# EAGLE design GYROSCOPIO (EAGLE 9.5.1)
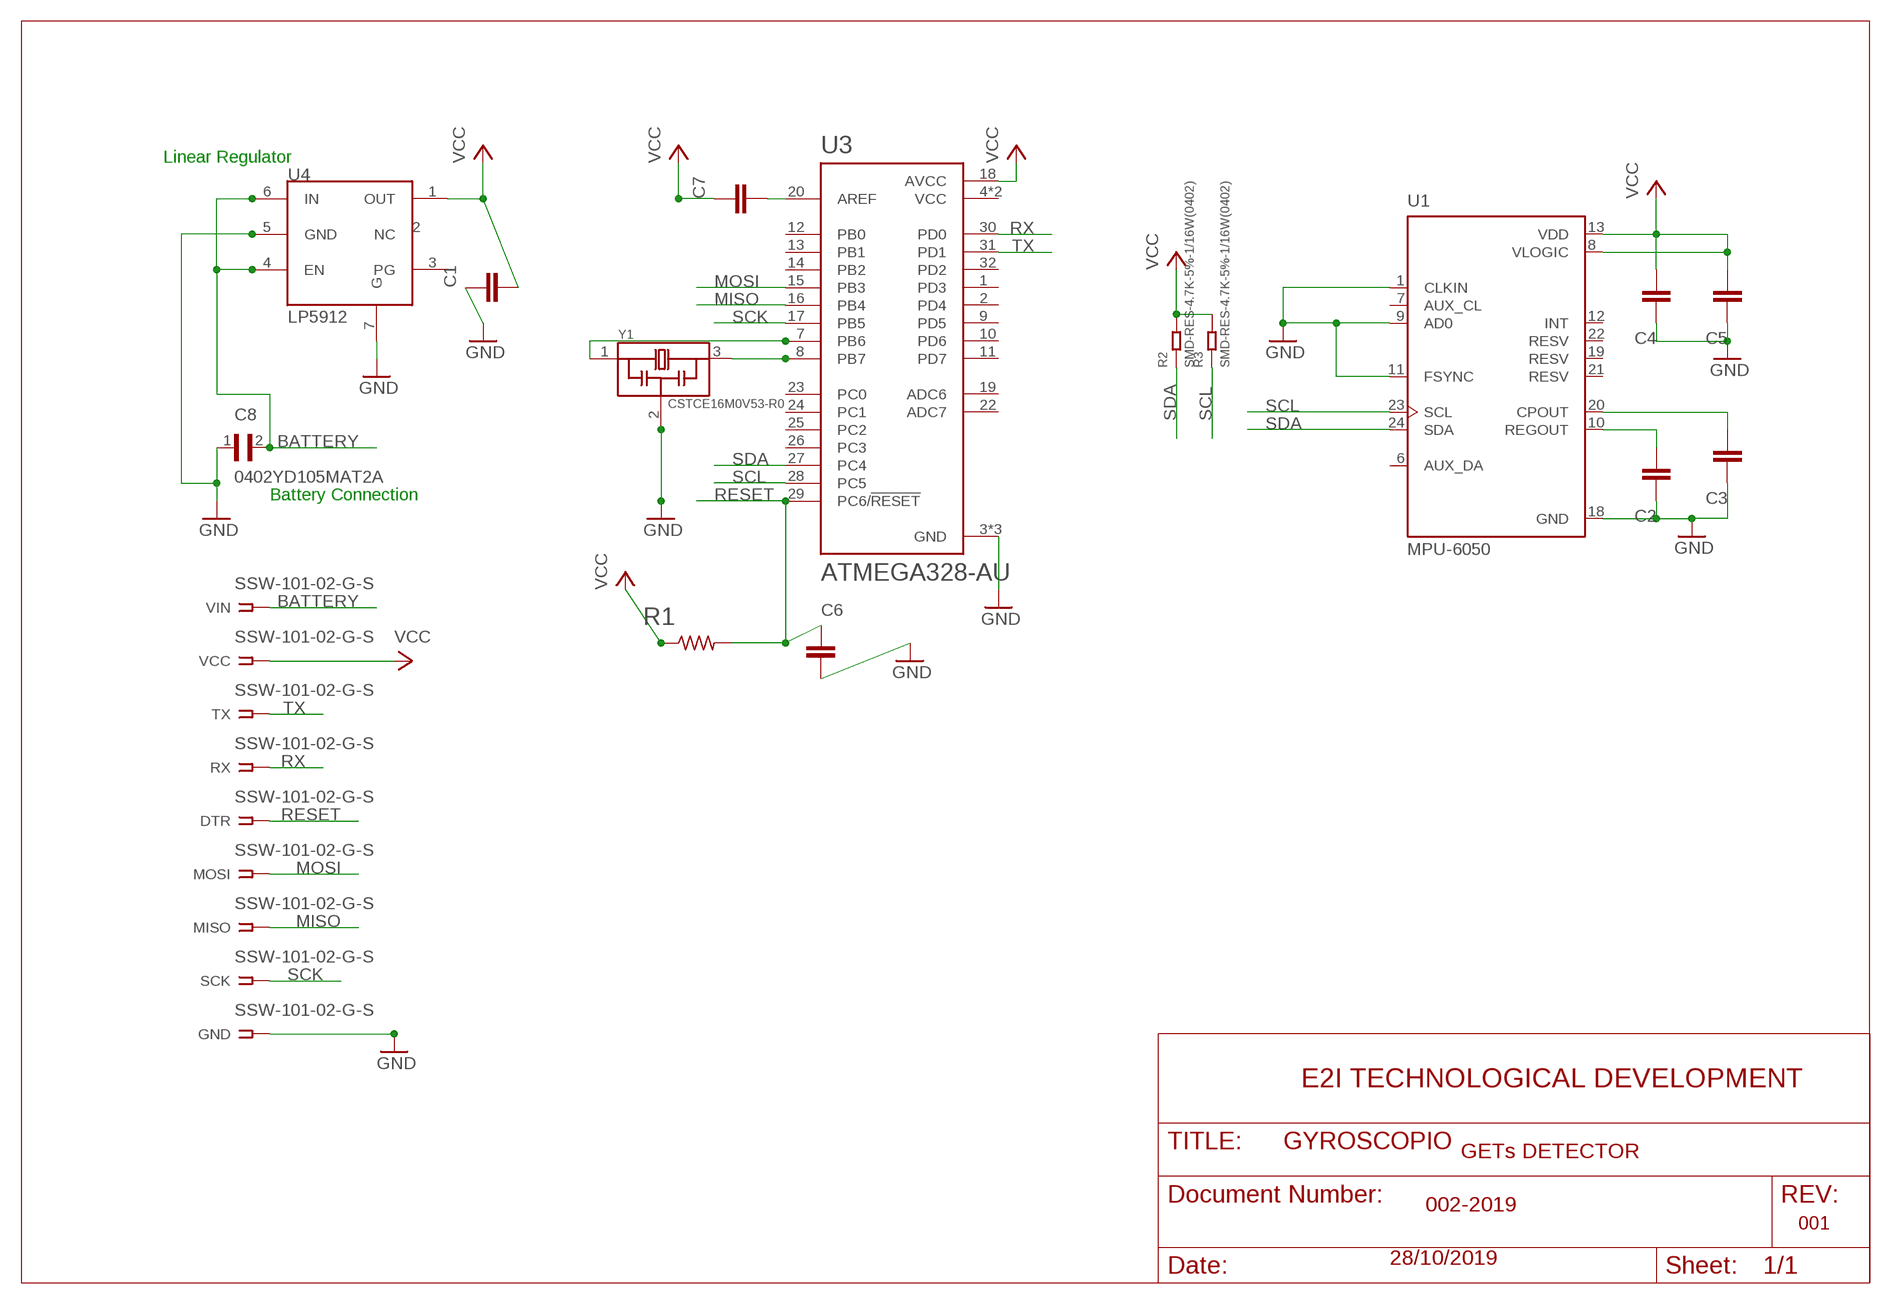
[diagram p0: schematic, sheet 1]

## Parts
C1  C-EUC0603  [C0603]
C2  C-EUC0603  [C0603]
C3  C-EUC0603  [C0603]
C4  C-EUC0603  [C0603]
C5  C-EUC0603  [C0603]
C6  C-EUC0603  [C0603]
C7  C-EUC0603  [C0603]
C8  0402YD105MAT2A  [CAPC1005X71N]
DTR  SSW-101-02-G-S  [SSW-101-02-G-S]
GND  SSW-101-02-G-S  [SSW-101-02-G-S]
MISO  SSW-101-02-G-S  [SSW-101-02-G-S]
MOSI  SSW-101-02-G-S  [SSW-101-02-G-S]
R1  R-US_R0603  [R0603]
R2  SMD-RES-4.7K-5%-1/16W(0402)  [R0402]
R3  SMD-RES-4.7K-5%-1/16W(0402)  [R0402]
RX  SSW-101-02-G-S  [SSW-101-02-G-S]
SCK  SSW-101-02-G-S  [SSW-101-02-G-S]
TX  SSW-101-02-G-S  [SSW-101-02-G-S]
U1  MPU-6050  [QFN50P400X400X95-24N]
U3  ATMEGA328-AU  [QFP80P900X900X120-32N]
U4  LP5912  [LP5912]
VCC  SSW-101-02-G-S  [SSW-101-02-G-S]
VIN  SSW-101-02-G-S  [SSW-101-02-G-S]
Y1  CSTCE16M0V53-R0  [OSC_CSTCE16M0V53-R0]

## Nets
BATTERY: C8.2 U4.4(EN) U4.6(IN) VIN.1
GND: C1.1 C2.1 C3.1 C4.1 C5.1 C6.2 C8.1 GND.1 U1.1(CLKIN) U1.9(AD0) U1.11(FSYNC) U1.18(GND) U3.3(GND) U3.5(GND) U3.21(GND) U4.5(GND) U4.7(G) Y1.2
MISO: MISO.1 U3.16(PB4)
MOSI: MOSI.1 U3.15(PB3)
N$1: U3.7(PB6) Y1.1
N$2: U3.8(PB7) Y1.3
N$3: C2.2 U1.10(REGOUT)
N$4: C3.2 U1.20(CPOUT)
N$11: C7.2 U3.20(AREF)
RESET: C6.1 DTR.1 R1.2 U3.29(PC6/!RESET)
RX: RX.1 U3.30(PD0)
SCK: SCK.1 U3.17(PB5)
SCL: R3.1 U1.23(SCL) U3.28(PC5)
SDA: R2.1 U1.24(SDA) U3.27(PC4)
TX: TX.1 U3.31(PD1)
VCC: C1.2 C4.2 C5.2 C7.1 R1.1 R2.2 R3.2 U1.8(VLOGIC) U1.13(VDD) U3.18(AVCC) U4.1(OUT) VCC.1
Unconnected: U1.6(AUX_DA) U1.7(AUX_CL) U1.12(INT) U1.19(RESV) U1.21(RESV) U1.22(RESV) U3.1(PD3) U3.2(PD4) U3.9(PD5) U3.10(PD6) U3.11(PD7) U3.12(PB0) U3.13(PB1) U3.14(PB2) U3.19(ADC6) U3.22(ADC7) U3.23(PC0) U3.24(PC1) U3.25(PC2) U3.26(PC3) U3.32(PD2) U4.2(NC) U4.3(PG)

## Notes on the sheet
- Linear Regulator
- Battery Connection
- E2I TECHNOLOGICAL DEVELOPMENT
- GETs DETECTOR
- 002-2019
- 001
- 28/10/2019

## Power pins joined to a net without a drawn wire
VCC: U3.4(VCC) U3.6(VCC)

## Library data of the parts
C1-C7 = rcl:C-EU: CAPACITOR, European symbol; SPICEPREFIX: C
C8 = Capacitor1uF:0402YD105MAT2A: CAP 1UF 16VDC X5R 20% SMD 0402; AVAILABILITY: Unavailable; DESCRIPTION: Cap 1uf 16vdc X5r 20% Smd 0402; MF: AVX; MP: 0402YD105MAT2A; PACKAGE: 1005 AVX; PRICE: None
DTR GND MISO MOSI RX SCK TX VCC VIN = con-samtec:SSW-101-02-G-S: THROUGH-HOLE .025" SQ POST SOCKET; MF: Samtec Inc.; MPN: SSW-101-02-G-S; OC_FARNELL: unknown; OC_NEWARK: 11P9336
R1 = rcl:R-US_: RESISTOR, American symbol; SPICEPREFIX: R
R2 R3 = RES-4.7K-SMD-5_-1_16W_0402_:SMD-RES-4.7K-5%-1/16W(0402): 301010010; AVAILABILITY: Unavailable; DESCRIPTION: Res Thick Film 0402 4.7K Ohm 5% 0.063W_1/16W_ ?100ppm/C Molded SMD Paper T/R; MF: Yageo; MP: RC0402JR074K7L; PACKAGE: 0402 Yageo; PRICE: None
U1 = MPU-6050:MPU-6050: MPU-6050 Six-Axis (Gyro + Accelerometer) MEMS MotionTracking™ Devices; AVAILABILITY: Unavailable; DESCRIPTION: 3-axis gyroscope, 3-axis accelerometer in a 4x4x0.9 housing; MF: TDK InvenSense; MP: MPU-6050; PACKAGE: QFN-24 InvenSense; PRICE: None
U3 = ATMEGA328-AU:ATMEGA328-AU: ATmega Series 20 MHz 32 KB Flash 2 KB SRAM 8-Bit Microcontroller - TQFP-32; AVAILABILITY: Unavailable; DESCRIPTION: ATmega Series 20 MHz 32 KB Flash 2 KB SRAM 8-Bit Microcontroller - TQFP-32; MF: Microchip; MP: ATMEGA328-AU; PACKAGE: TQFP-32 Microchip; PRICE: None
U4 = electronic-labs:LP5912
Y1 = CSTCE16M0V53-R0:CSTCE16M0V53-R0: 16MHz Ceramic Resonator Built in Capacitor 15pF ±0.3% -20°C ~ 80°C Surface Mount; AVAILABILITY: Unavailable; DESCRIPTION: Ceramic Resonator 16MHz ??0.5% _Tol_ ??0.3% _Stability_ 15pF 40Ohm 3-Pin CSMD T/R; MF: Murata; MP: CSTCE16M0V53-R0; PACKAGE: SMD-3 Murata; PRICE: None

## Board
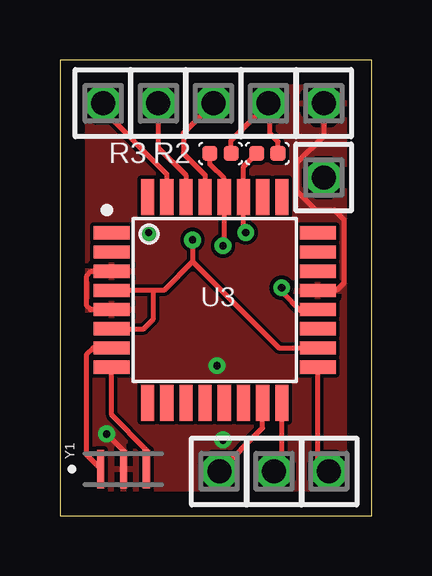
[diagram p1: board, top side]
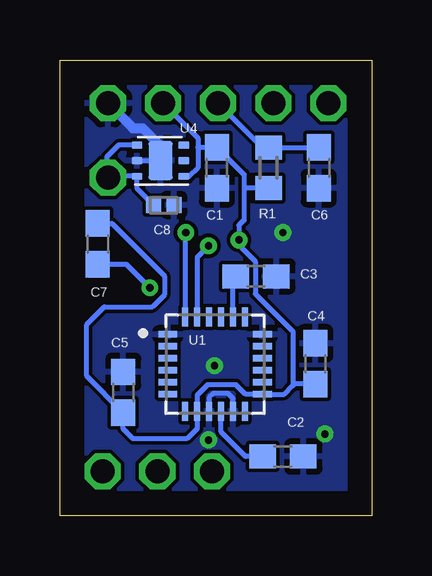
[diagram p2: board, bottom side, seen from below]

Size 13 x 19 mm. Coordinates in mm from the lower left corner, seen from the top.
Outline: 0,0 13,0 13,19 0,19 0,0
Copper layers (1*16): Top 0.035mm / dielectric 1.5mm / Bottom 0.035mm
Design rules "default *": minimum track width 6mil, minimum drill 0.3mm, track to track 6mil, track to pad 6mil, pad to pad 6mil, via to via 6mil, smd to smd 6mil, copper to edge 40mil, drill to drill 6mil, minimum pad ring 10mil, minimum via ring 8mil, stop-mask expansion 4mil, vias tented up to drill 0.5mm, thermal gap 10mil

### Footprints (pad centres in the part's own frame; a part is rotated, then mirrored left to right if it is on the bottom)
C0603 = smd 1.1 x 1: 1 -0.85,0; 2 0.85,0
CAPC1005X71N = smd 0.62 x 0.67: 1 -0.425,0; 2 0.425,0
SSW-101-02-G-S = drill 1 pad 1.5 octagon: 1 0,0
R0603 = smd 1 x 1.1: 1 -0.85,0; 2 0.85,0
R0402 = smd 0.635 x 0.635: 1 0,0.445; 2 0,-0.445
QFN50P400X400X95-24N = smd 0.79 x 0.26: 1 -1.97,1.25; 2 -1.97,0.75; 3 -1.97,0.25; 4 -1.97,-0.25; 5 -1.97,-0.75; 6 -1.97,-1.25; 13 1.97,-1.25; 14 1.97,-0.75; 15 1.97,-0.25; 16 1.97,0.25; 17 1.97,0.75; 18 1.97,1.25 | smd 0.26 x 0.79: 7 -1.25,-1.97; 8 -0.75,-1.97; 9 -0.25,-1.97; 10 0.25,-1.97; 11 0.75,-1.97; 12 1.25,-1.97; 19 1.25,1.97; 20 0.75,1.97; 21 0.25,1.97; 22 -0.25,1.97; 23 -0.75,1.97; 24 -1.25,1.97
QFP80P900X900X120-32N = smd 1.5 x 0.55: 1 -4.3,2.8; 2 -4.3,2; 3 -4.3,1.2; 4 -4.3,0.4; 5 -4.3,-0.4; 6 -4.3,-1.2; 7 -4.3,-2; 8 -4.3,-2.8; 17 4.3,-2.8; 18 4.3,-2; 19 4.3,-1.2; 20 4.3,-0.4; 21 4.3,0.4; 22 4.3,1.2; 23 4.3,2; 24 4.3,2.8 | smd 0.55 x 1.5: 9 -2.8,-4.3; 10 -2,-4.3; 11 -1.2,-4.3; 12 -0.4,-4.3; 13 0.4,-4.3; 14 1.2,-4.3; 15 2,-4.3; 16 2.8,-4.3; 25 2.8,4.3; 26 2,4.3; 27 1.2,4.3; 28 0.4,4.3; 29 -0.4,4.3; 30 -1.2,4.3; 31 -2,4.3; 32 -2.8,4.3
LP5912 = smd 0.45 x 0.3: 1 0,0.65; 2 0,0; 3 0,-0.65; 4 1.95,-0.65; 5 1.95,0; 6 1.95,0.65 | smd 1 x 1.6: 7 0.975,0
OSC_CSTCE16M0V53-R0 = smd 0.3 x 1.6: 1 -0.95,0; 2 0,0; 3 0.95,0

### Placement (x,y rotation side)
C1  6.45,14.5 90 bottom
C2  3.7,2.46 180 bottom
C3  4.82,9.98 180 bottom
C4  2.35,6.33 270 bottom
C5  10.36,5.14 270 bottom
C6  2.2,14.5 270 bottom
C7  11.42,11.33 270 bottom
C8  8.67,12.95 180 bottom
DTR  6.4,17.2 270 top
GND  11,17.2 270 top
MISO  8.94,1.84 90 top
MOSI  6.65,1.84 90 top
R1  4.3,14.5 90 bottom
R2  8.65,15.1 90 top
R3  6.7,15.1 90 top
RX  4.1,17.2 270 top
SCK  11.22,1.84 90 top
TX  1.8,17.2 270 top
U1  6.53,6.31 0 bottom
U3  6.46,8.99 0 top
U4  7.83,14.8 180 bottom
VCC  8.7,17.2 270 top
VIN  11,14.1 270 top
Y1  2.65,1.94 0 top

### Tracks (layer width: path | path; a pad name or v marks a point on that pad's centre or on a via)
BATTERY
  Bottom 0.2: U4.4 10.55,15.45 11.05,14.95 11.05,14.15 VIN.1 10.95,14.15 U4.6 9.78,13.63 C8.2
GND  (via drill 0.3)
  Top 0.2: Y1.2 2.65,2.7 v1.95,3.4 | U3.5 1.28,8.59 1.12,8.75 1.12,10 1.31,10.19 U3.3 | GND.1 11,15.82 9.89,14.72 9.89,13.53 10.68,12.74 11.46,12.74 11.85,12.35 11.85,9.7 11.54,9.39 U3.21
  Bottom 0.2: U4.5 U4.7 | U1.11 5.78,4.88 6,5.1 6.6,5.1 6.78,4.92 U1.9
  Bottom 0.406: GND.1 9.95,16.15 9.55,16.15 8.8,15.4 U4.7
  other vias: 6.55,6.25 3.7,11.8 6.8,3.15
  pour Bottom: 0.3,18.7 0.3,0.3 12.6,0.3 12.6,18.7
  pour Top: 0.05,18.85 12.9,18.85 12.9,0.1 0.05,0.1
MISO
  Top 0.2: MISO.1 9.26,2.16 U3.16
MOSI
  Top 0.2: MOSI.1 8.46,3.65 U3.15
N$1
  Top 0.2: Y1.1 1.12,2.52 1.12,6.73 1.38,6.99 U3.7
N$2
  Top 0.2: Y1.3 3.6,2.75 2.16,4.19 U3.8
N$3
  Bottom 0.2: U1.10 6.28,3.48 5.26,2.46 C2.2
N$4
  Bottom 0.2: U1.20 5.78,9.98 C3.2
N$11  (via drill 0.3)
  Top 0.2: U3.20 10.67,8.5 10.1,8.5 9.25,9.35 v9.25,9.5
  Bottom 0.2: C7.2 10.23,10.48 v9.25,9.5
RESET
  Top 0.2: DTR.1 5.15,15.95 5.15,15.1 6.06,14.19 U3.29
  Bottom 0.2: C6.1 R1.2 4.43,15.23 DTR.1
RX
  Top 0.2: RX.1 4.1,15.35 5.26,14.19 U3.30
SCK
  Top 0.2: SCK.1 10.76,2.3 U3.17
SCL  (via drill 0.3)
  Top 0.2: v6.8,11.25 6.86,11.31 U3.28 6.86,14.04 6.25,14.64 R3.1
  Bottom 0.2: v6.8,11.25 7.28,10.77 U1.23
SDA  (via drill 0.3)
  Top 0.2: R2.1 7.66,14.55 U3.27 7.66,11.89 v7.75,11.8
  Bottom 0.2: v7.75,11.8 7.78,11.77 U1.24
TX
  Top 0.2: TX.1 1.8,16.9 4.46,14.24 U3.31
VCC  (via drill 0.3)
  Top 0.2: R3.2 7.14,15.64 VCC.1 8.74,17.16 8.74,15.95 9.1,15.6 R2.2 | v5.54,11.5 5.54,10.59 | 3.85,9.39 4.34,9.39 5.54,10.59 | 3.85,9.39 U3.4 | U3.6 3.49,7.79 3.9,8.2 3.9,9.34 3.85,9.39 | 5.54,10.59 9.13,6.99 U3.18
  Bottom 0.2: VCC.1 7.25,15.75 7.25,15.35 | 7.25,15.35 7.25,14.5 7.6,14.15 U4.1 | C4.2 3.22,5.48 3.27,5.42 | 3.27,5.42 3.64,5.06 U1.13 5.26,5.06 5.65,5.45 6.85,5.45 7.28,5.02 U1.8 7.28,3.62 7.7,3.2 9.95,3.2 10.36,3.61 C5.2 11.88,5.81 11.88,7.97 11.15,8.7 9.14,8.7 8.64,9.2 8.64,9.99 10.83,12.18 C7.1 | 7.25,15.35 C1.2 5.32,14.22 5.32,13.65 | 3.27,5.42 3.27,7.67 4.85,9.25 4.85,10.6 5.54,11.29 v5.54,11.5 5.54,12.11 5.32,12.32 5.32,13.65 | R1.1 5.32,13.65

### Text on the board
bNames: U4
